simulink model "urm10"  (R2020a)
settings: Solver=VariableStepAuto  StartTime=0.0  StopTime=inf  RelTol=1e-3
model workspace (MAT data in the model file):
  rp_cyclique_esp = 20

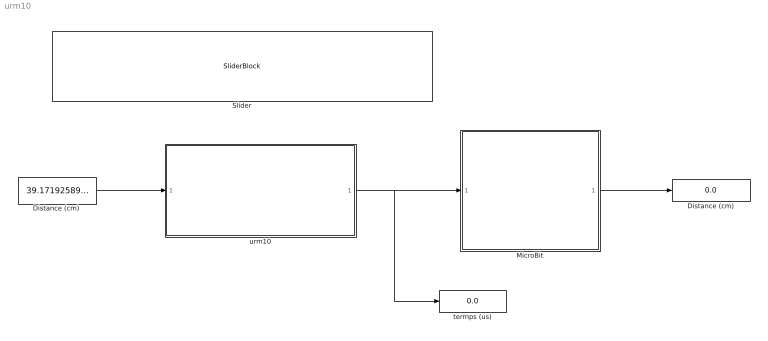
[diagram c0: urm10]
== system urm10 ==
  Distance (cm) : Display
  "Distance (cm) " : Constant  Value=39.17192589576548
  MicroBit : Subsystem
  Slider : SliderBlock  ScaleMax=50  TickInterval=10
  termps (us) : Display
  urm10 : Subsystem
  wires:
  "Distance (cm) "/1 -> urm10/1(In1)
  urm10/1(Out1) -> termps (us)/1, MicroBit/1(In1)
  MicroBit/1(Out1) -> Distance (cm)/1

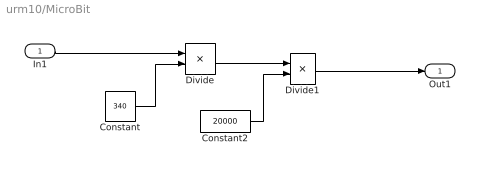
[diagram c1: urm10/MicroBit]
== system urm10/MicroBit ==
  In1 : Inport
  Constant : Constant  Value=340
  Constant2 : Constant  Value=20000
  Divide : Product  Inputs=**
  Divide1 : Product  Inputs=*/
  Out1 : Outport  VectorParamsAs1DForOutWhenUnconnected=off
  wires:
  Divide1/1 -> Out1/1
  In1/1 -> Divide/1
  Constant/1 -> Divide/2
  Divide/1 -> Divide1/1
  Constant2/1 -> Divide1/2

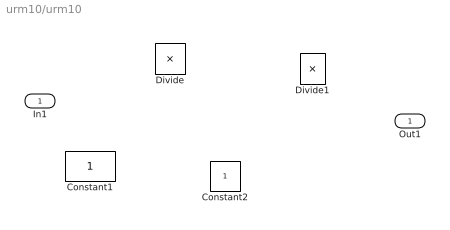
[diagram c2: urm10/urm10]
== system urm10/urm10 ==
  In1 : Inport
  Constant1 : Constant
  Constant2 : Constant
  Divide : Product  Inputs=**
  Divide1 : Product  Inputs=*/
  Out1 : Outport  VectorParamsAs1DForOutWhenUnconnected=off
